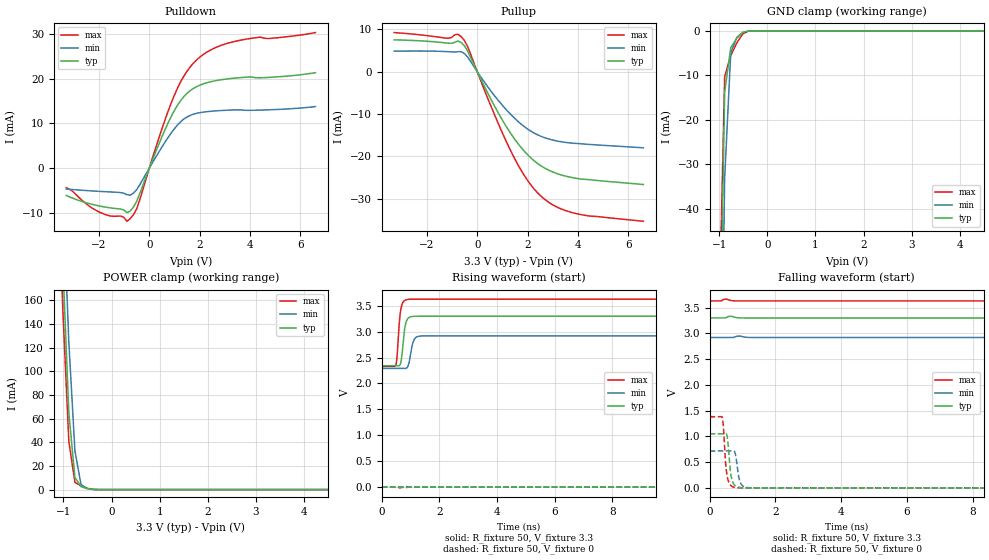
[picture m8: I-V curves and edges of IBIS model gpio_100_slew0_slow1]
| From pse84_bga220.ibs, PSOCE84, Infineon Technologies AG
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[Model] gpio_100_slew0_slow1
Model_type I/O
Enable   Active-High
Vinl  =  0.99
Vinh  =  2.31
Vmeas =  1.65
Cref  =  15e-12
| Capacitance   typ   min   max
C_comp   1.09946e-12   1.08623e-12   1.11440e-12
| Variables   typ   min   max
[GND Clamp Reference]   0   0   0
[POWER Clamp Reference]   3.3   2.92   3.63
[Pulldown Reference]   0   0   0
[Pullup Reference]   3.3   2.92   3.63
[Temperature Range]   25   125   -40
[Voltage Range]   3.3   2.92   3.63
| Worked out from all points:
|   slope of the pulldown table from 0 to 0.495 V, typ, clamps not added: 71.6 ohm
|   slope of the pullup table from 0 to 0.495 V, typ, clamps not added: 83.3 ohm
|   GND clamp passes 1 mA (typ) near -0.57 V on its own axis
|   POWER clamp passes 1 mA (typ) near -0.52 V on its own axis
|   falling waveform, R_fixture 50, V_fixture 3.3: 20-80 % time 694ns typ, 1.01us min, 397ns max; typ from 3.3 V to 2.34 V
|   falling waveform, R_fixture 50, V_fixture 0: 20-80 % time 96.8ps typ, 105ps min, 93.7ps max; typ from 1.05 V to 0 V
|   rising waveform, R_fixture 50, V_fixture 3.3: 20-80 % time 114ps typ, 134ps min, 103ps max; typ from 2.34 V to 3.3 V
|   rising waveform, R_fixture 50, V_fixture 0: 20-80 % time 754ns typ, 1.06us min, 488ns max; typ from 0 V to 1.04 V
[GND Clamp]
| Voltage   I(typ)   I(min)   I(max)
-1.65V    -892.5mA   -911.9mA   -883.9mA
-1.015V   -92.32mA   -129.7mA   -71.28mA
-888.3mV  -13.83mA   -33.21mA   -10.31mA
-761.4mV  -3.792mA   -4.944mA   -5.509mA
-634.5mV  -1.622mA   -1.436mA   -2.707mA
-507.6mV  -326.2uA   -352.3uA   -651.6uA
-380.7mV  -13.48uA   -32.14uA   -19.55uA
-253.8mV  -189.4nA   -1.276uA   -466.7nA
6.6V      0A         0A         0A
[POWER Clamp]
| Voltage   I(typ)   I(min)   I(max)
-1.523V   838.1mA    872.9mA    823.9mA
-1.142V   346.5mA    405.1mA    310.5mA
-1.015V   193mA      257.4mA    153.9mA
-888.3mV  64.97mA    124.9mA    40.96mA
-761.4mV  10.28mA    32.7mA     6.184mA
-634.5mV  2.553mA    4.346mA    3.067mA
-507.6mV  805.9uA    960.7uA    1.159mA
-253.8mV  1.454uA    10.02uA    1.678uA
6.6V      0A         0A         0A
[Pulldown]
| Voltage   I(typ)   I(min)   I(max)
-3.3V     -6.15mA    -4.695mA   -4.423mA
-2.157V   -8.273mA   -5.161mA   -9.338mA
-1.142V   -9.173mA   -5.494mA   -10.74mA
-888.3mV  -9.988mA   -5.953mA   -11.91mA
-507.6mV  -7.509mA   -4.873mA   -9.177mA
341.4mV   4.84mA     3.249mA    6.058mA
910.3mV   11.98mA    8.158mA    15.13mA
1.366V    15.94mA    10.93mA    20.51mA
1.821V    18.03mA    12.15mA    23.86mA
2.503V    19.39mA    12.72mA    26.59mA
3.3V      20.06mA    12.98mA    28.19mA
6.6V      21.33mA    13.74mA    30.3mA
[Pullup]
| Voltage   I(typ)   I(min)   I(max)
-3.3V     7.527mA    4.862mA    9.247mA
-1.142V   6.736mA    4.723mA    7.893mA
-761.4mV  7.259mA    4.727mA    8.836mA
-634.5mV  6.867mA    4.72mA     8.248mA
-380.7mV  4.868mA    3.47mA     5.906mA
682.8mV   -8.07mA    -5.639mA   -10.11mA
1.479V    -15.86mA   -10.96mA   -20.44mA
2.048V    -19.88mA   -13.73mA   -26.08mA
2.731V    -22.92mA   -15.68mA   -30.37mA
3.3V      -24.31mA   -16.5mA    -32.32mA
4.051V    -25.28mA   -16.98mA   -33.65mA
6.6V      -26.63mA   -17.96mA   -35.32mA
[Ramp]
dV/dt_r   0.625855/0.754303u  0.420963/1.05906u  0.82799/0.488121u
dV/dt_f   0.573974/0.693926u  0.373545/1.0113u  0.781638/0.397251u
R_load = 50
[Falling Waveform]
R_fixture = 50
V_fixture = 3.3
V_fixture_min = 2.92
V_fixture_max = 3.63
| Time   V(typ)   V(min)   V(max)
0s        3.3V       2.92V      3.63V
506.1ps   3.308V     2.92V      3.665V
135.4ns   3.3V       2.92V      3.582V
310.1ns   3.199V     2.916V     3.047V
473ns     2.976V     2.865V     2.729V
635.9ns   2.797V     2.77V      2.56V
880.2ns   2.62V      2.638V     2.441V
1.285us   2.471V     2.492V     2.368V
1.917us   2.386V     2.379V     2.336V
4us       2.343V     2.297V     2.327V
[Falling Waveform]
R_fixture = 50
V_fixture = 0
V_fixture_min = 0
V_fixture_max = 0
| Time   V(typ)   V(min)   V(max)
0s        1.049V     715.2mV    1.381V
383ps     1.049V     715.1mV    1.365V
416.2ps   1.049V     715.1mV    1.199V
511.4ps   1.041V     715.2mV    314mV
627.2ps   335mV      715.3mV    58.38mV
677.9ps   154.2mV    715.9mV    28.33mV
775.5ps   39.72mV    672.4mV    7.438mV
888.1ps   8.979mV    199.3mV    1.148mV
973.6ps   2.291mV    58.96mV    385.4uV
4us       19.97nV    549.4nV    10.01nV
[Rising Waveform]
R_fixture = 50
V_fixture = 3.3
V_fixture_min = 2.92
V_fixture_max = 3.63
| Time   V(typ)   V(min)   V(max)
0s        2.342V     2.29V      2.327V
481.1ps   2.341V     2.29V      2.345V
624.9ps   2.351V     2.29V      3.273V
684.1ps   2.475V     2.29V      3.491V
830.5ps   3.157V     2.29V      3.614V
932.9ps   3.269V     2.373V     3.626V
1.064ns   3.294V     2.752V     3.629V
1.35ns    3.299V     2.916V     3.629V
5.098ns   3.3V       2.92V      3.63V
4us       3.3V       2.92V      3.63V
[Rising Waveform]
R_fixture = 50
V_fixture = 0
V_fixture_min = 0
V_fixture_max = 0
| Time   V(typ)   V(min)   V(max)
0s        17.41nV    537.5nV    10.27nV
144.3ns   988.3uV    73uV       55.28mV
250.6ns   41.54mV    2.216mV    313.5mV
398.7ns   203.4mV    33.71mV    673.2mV
561.6ns   402.2mV    111.2mV    944.7mV
724.5ns   569.4mV    203mV      1.104V
968.8ns   747.1mV    331.9mV    1.223V
1.364us   896.6mV    485.6mV    1.309V
2.003us   986.8mV    612.8mV    1.358V
4us       1.043V     701.6mV    1.38V
